TYPE STR_BPG400 :
STRUCT
	Combination_Gauge_Reading_Valid_Module_1		:	BIT	;
	Combination_Gauge_Overrange_Exceeded_Module_1	:	BIT	;
	Combination_Gauge_Underrange_Exceeded_Module_1	:	BIT	;
	Combination_Gauge_Active_Value_Module_1			:	REAL	;
	Combination_Gauge_Active_Sensor_Number_Module_1	:	UINT	;
	Combination_Gauge_Reading_Valid_Module_2		:	BIT	;
	Combination_Gauge_Overrange_Exceeded_Module_2	:	BIT	;
	Combination_Gauge_Underrange_Exceeded_Module_2	:	BIT	;
	Combination_Gauge_Active_Value_Module_2			:	REAL	;
	Combination_Gauge_Active_Sensor_Number_Module_2	:	UINT	;
	Active_Exception_Status							:	USINT	;
	Trip_Point_Output_All_Instance					:	UDINT	;
	WcState											:	BIT	;
	InputToggle										:	BIT	;
	State											:	UINT	;
	//AdsAddr										:	AMSADDR	;

END_STRUCT
END_TYPE
